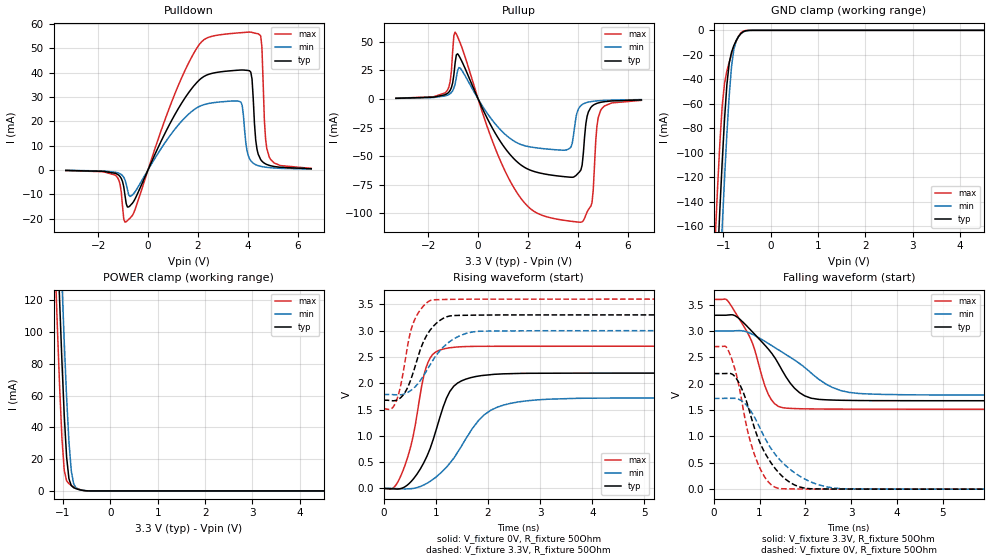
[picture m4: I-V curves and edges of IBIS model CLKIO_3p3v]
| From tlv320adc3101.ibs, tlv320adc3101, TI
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|   CLKIO_3p3v
[Model]   CLKIO_3p3v
Model_type   I/O
Polarity   Non-Inverting
Enable   Active-High
Vinl = 0.99
Vinh = 2.31
Vmeas = 1.65
Vref = 0
Cref = 5pF
Rref = 1000000
|   typ   min   max
C_comp   1.630pF   1.592pF   1.693pF
[Voltage Range]   3.3   3   3.6
[Temperature Range]   27   85   -40
[Pullup Reference]   3.3   3   3.6
[Pulldown Reference]   -0   -0   -0
[Power Clamp Reference]   3.3   3   3.6
[GND Clamp Reference]   -0   -0   -0
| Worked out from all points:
|   slope of the pulldown table from 0 to 0.495 V, typ, clamps not added: 44.4 ohm
|   slope of the pullup table from 0 to 0.495 V, typ, clamps not added: 22.1 ohm
|   GND clamp passes 1 mA (typ) near -0.57 V on its own axis
|   POWER clamp passes 1 mA (typ) near -0.68 V on its own axis
|   falling waveform, V_fixture 3.3V, R_fixture 50Ohm: 20-80 % time 825ps typ, 1.18ns min, 537ps max; typ from 3.3 V to 1.68 V
|   rising waveform, V_fixture 0V, R_fixture 50Ohm: 20-80 % time 482ps typ, 761ps min, 333ps max; typ from 0 V to 2.19 V
|   rising waveform, V_fixture 3.3V, R_fixture 50Ohm: 20-80 % time 373ps typ, 536ps min, 264ps max; typ from 1.68 V to 3.3 V
|   falling waveform, V_fixture 0V, R_fixture 50Ohm: 20-80 % time 621ps typ, 829ps min, 441ps max; typ from 2.19 V to 0 V
[Pulldown]
|   Voltage   I(typ)   I(min)   I(max)
-3.3V     -212.1uA   -165.3uA   -254.8uA
-1.32V    -1.377mA   -921.5uA   -2.121mA
-874.5mV  -13.95mA   -5.813mA   -21.28mA
1.996V    36.36mA    25.76mA    50.68mA
3.729V    41.1mA     27.9mA     56.46mA
4.075V    40.77mA    4.614mA    56.7mA
4.175V    37.43mA    3.189mA    56.58mA
4.323V    12.2mA     2.145mA    56.19mA
4.521V    4.257mA    1.479mA    55.18mA
4.719V    2.469mA    1.124mA    12.64mA
4.867V    1.865mA    951.1uA    5.256mA
6.551V    483.1uA    342.9uA    619.7uA
[GND Clamp]
|   Voltage   I(typ)   I(min)   I(max)
-3.3V     -2.298A    -2.352A    -2.242A
-1.171V   -232.7mA   -290.4mA   -171.9mA
-1.122V   -189.3mA   -246.3mA   -130.6mA
-1.073V   -147.6mA   -203.2mA   -92.89mA
-1.023V   -108.2mA   -161.5mA   -62.34mA
-973.5mV  -72.97mA   -121.8mA   -43.41mA
-924mV    -44.76mA   -85.16mA   -33.42mA
-874.5mV  -26.9mA    -53.49mA   -26.15mA
-825mV    -17.81mA   -29.61mA   -19.66mA
-726mV    -8.325mA   -8.566mA   -8.713mA
-577.5mV  -1.124mA   -1.328mA   -644.8uA
6.551V    0A         0A         0A
[Pullup]
|   Voltage   I(typ)   I(min)   I(max)
-3.3V     578.7uA    490.1uA    654.5uA
-1.32V    3.716mA    2.675mA    5.338mA
-1.122V   7.589mA    4.666mA    15.39mA
-924mV    31.57mA    13.21mA    58.48mA
-726mV    36.02mA    27.09mA    49.2mA
1.551V    -54.69mA   -38.18mA   -81.66mA
3.63V     -68.27mA   -43.76mA   -106.6mA
4.075V    -63.55mA   -6.996mA   -107.7mA
4.571V    -6.292mA   -2.155mA   -90.51mA
4.769V    -3.838mA   -1.671mA   -23.59mA
4.917V    -2.953mA   -1.428mA   -9.995mA
6.551V    -815.9uA   -544uA     -1.216mA
[POWER Clamp]
|   Voltage   I(typ)   I(min)   I(max)
-3.3V     2.271A     2.32A      2.221A
-1.171V   205.7mA    259.8mA    148mA
-1.122V   162.4mA    216mA      105.8mA
-1.073V   120.8mA    173.4mA    66.54mA
-1.023V   81.86mA    132.4mA    33.49mA
-973.5mV  47.46mA    93.85mA    12.96mA
-924mV    21.38mA    59.14mA    6.364mA
-874.5mV  7.678mA    30.9mA     4.556mA
-825mV    3.346mA    12.57mA    3.514mA
-775.5mV  2.05mA     4.501mA    2.646mA
-726mV    1.411mA    1.926mA    1.884mA
6.551V    0A         0A         0A
[Ramp]
R_load = 50
|   typ   min   max
dV/dt_r   1.31543/4.82292e-010   1.03267/7.6132e-010   1.62415/3.32554e-010
dV/dt_f   0.973384/8.24834e-010  0.728766/1.18393e-009   1.24965/5.37229e-010
[Falling Waveform]
V_fixture = 3.3V
V_fixture_min = 3V
V_fixture_max = 3.6V
R_fixture = 50Ohm
C_fixture = 0F
|   Time   V(typ)   V(min)   V(max)
0s        3.3V       3V         3.6V
260.2ps   3.3V       3V         3.605V
382.4ps   3.309V     3.001V     3.476V
812.6ps   3.013V     2.951V     2.836V
1.185ns   2.662V     2.767V     1.807V
1.509ns   2.228V     2.59V      1.544V
1.984ns   1.771V     2.309V     1.524V
2.441ns   1.696V     1.997V     1.52V
2.946ns   1.685V     1.837V     1.519V
8.32ns    1.678V     1.785V     1.517V
[Rising Waveform]
V_fixture = 0V
V_fixture_min = 0V
V_fixture_max = 0V
R_fixture = 50Ohm
C_fixture = 0F
|   Time   V(typ)   V(min)   V(max)
0s        356uV      27.86uV    -1.161mV
272.9ps   -11.46mV   -3.963mV   125.7mV
575.6ps   187.4mV    1.63mV     1.046V
812.6ps   576.5mV    88.76mV    2.297V
1.116ns   1.47V      314.4mV    2.643V
1.268ns   1.842V     479.4mV    2.674V
1.497ns   2.047V     813.5mV    2.694V
1.939ns   2.152V     1.408V     2.702V
2.441ns   2.182V     1.619V     2.702V
8.32ns    2.193V     1.721V     2.706V
[Rising Waveform]
V_fixture = 3.3V
V_fixture_min = 3V
V_fixture_max = 3.6V
R_fixture = 50Ohm
C_fixture = 0F
|   Time   V(typ)   V(min)   V(max)
0s        1.678V     1.785V     1.516V
234.8ps   1.674V     1.78V      1.643V
400ps     1.811V     1.798V     2.356V
489.5ps   1.988V     1.843V     2.871V
564.8ps   2.198V     1.897V     3.138V
764.5ps   2.794V     2.143V     3.47V
895.2ps   3.015V     2.357V     3.574V
1.347ns   3.287V     2.846V     3.596V
1.821ns   3.295V     2.987V     3.598V
8.32ns    3.3V       3V         3.6V
[Falling Waveform]
|Gnd
V_fixture = 0V
V_fixture_min = 0V
V_fixture_max = 0V
R_fixture = 50Ohm
C_fixture = 0F
|   Time   V(typ)   V(min)   V(max)
0s        2.193V     1.721V     2.706V
272.9ps   2.195V     1.723V     2.696V
485ps     2.108V     1.72V      2.202V
730ps     1.621V     1.577V     1.135V
853.9ps   1.256V     1.42V      744.6mV
1.06ns    783.3mV    1.066V     305.4mV
1.324ns   410.6mV    679.7mV    41.26mV
1.872ns   42.34mV    249.5mV    3.762mV
2.588ns   3.262mV    25.18mV    1.537mV
8.32ns    -982.4nV   21.15uV    -6.042uV
